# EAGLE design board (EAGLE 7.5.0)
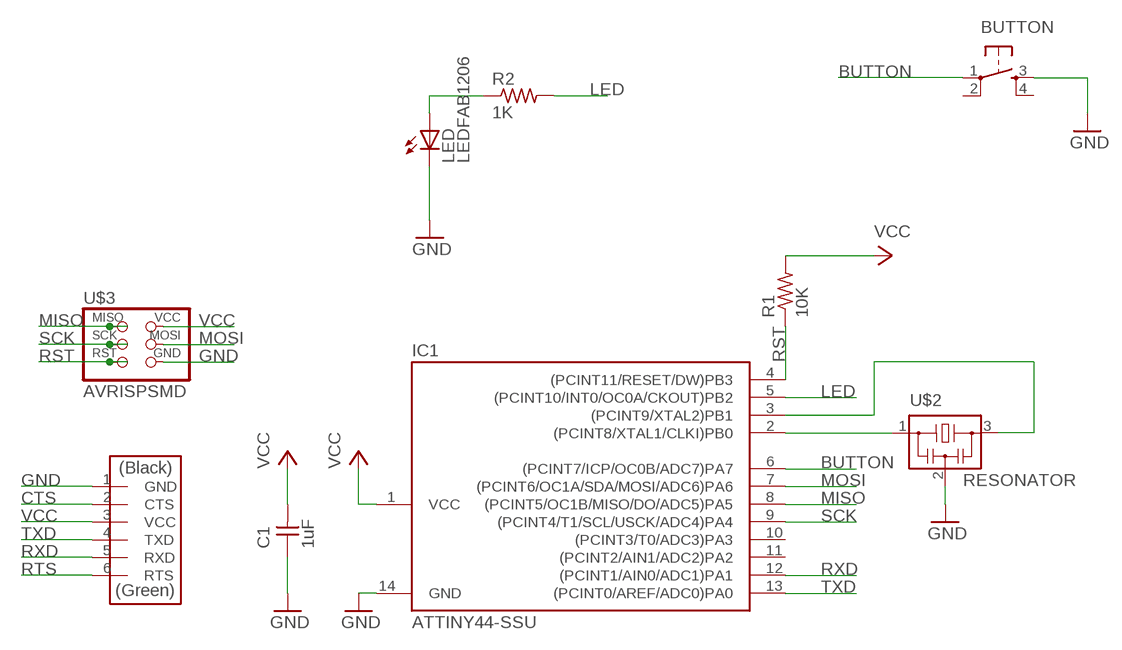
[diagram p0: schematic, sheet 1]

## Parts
BUTTON  6MM_SWITCH6MM_SWITCH  [6MM_SWITCH]
C1  1uF  CAP-UNPOLARIZED  [C1206]
IC1  ATTINY44-SSU  [SOIC14]
LED  LEDFAB1206  [LED1206FAB]
R1  10K  RES-US1206FAB  [R1206FAB]
R2  1K  RES-US1206FAB  [R1206FAB]
U$2  RESONATOR  [EFOBM]
U$3  AVRISPSMD  [2X03SMD]
U$4  FTDI-SMD-HEADER  [1X06SMD]

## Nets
BUTTON: BUTTON.1(P) IC1.6((PCINT7/ICP/OC0B/ADC7)PA7)
CTS: U$4.2(CTS)
GND: BUTTON.3(S) C1.1 IC1.14(GND) LED.2(C) U$2.2 U$3.6(GND) U$4.1(GND)
LED: IC1.5((PCINT10/INT0/OC0A/CKOUT)PB2) R2.2
MISO: IC1.8((PCINT5/OC1B/MISO/DO/ADC5)PA5) U$3.1(MISO)
MOSI: IC1.7((PCINT6/OC1A/SDA/MOSI/ADC6)PA6) U$3.4(MOSI)
N$1: IC1.3((PCINT9/XTAL2)PB1) U$2.3
N$2: IC1.2((PCINT8/XTAL1/CLKI)PB0) U$2.1
N$3: LED.1(A) R2.1
RST: IC1.4((PCINT11/RESET/DW)PB3) R1.1 U$3.5(RST)
RTS: U$4.6(RTS)
RXD: IC1.12((PCINT1/AIN0/ADC1)PA1) U$4.5(RXD)
SCK: IC1.9((PCINT4/T1/SCL/USCK/ADC4)PA4) U$3.3(SCK)
TXD: IC1.13((PCINT0/AREF/ADC0)PA0) U$4.4(TXD)
VCC: C1.2 IC1.1(VCC) R1.2 U$3.2(VCC) U$4.3(VCC)
Unconnected: BUTTON.2(P1) BUTTON.4(S1) IC1.10((PCINT3/T0/ADC3)PA3) IC1.11((PCINT2/AIN1/ADC2)PA2)

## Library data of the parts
BUTTON = fab:6MM_SWITCH: OMRON SWITCH
C1 = fab:CAP-UNPOLARIZED
IC1 = fab:ATTINY44
LED = fab:LED: LED
R1 R2 = fab:RES-US: Resistor (US Symbol)
U$2 = fab:RESONATOR
U$3 = fab:AVRISP
U$4 = fab:FTDI-SMD-HEADER

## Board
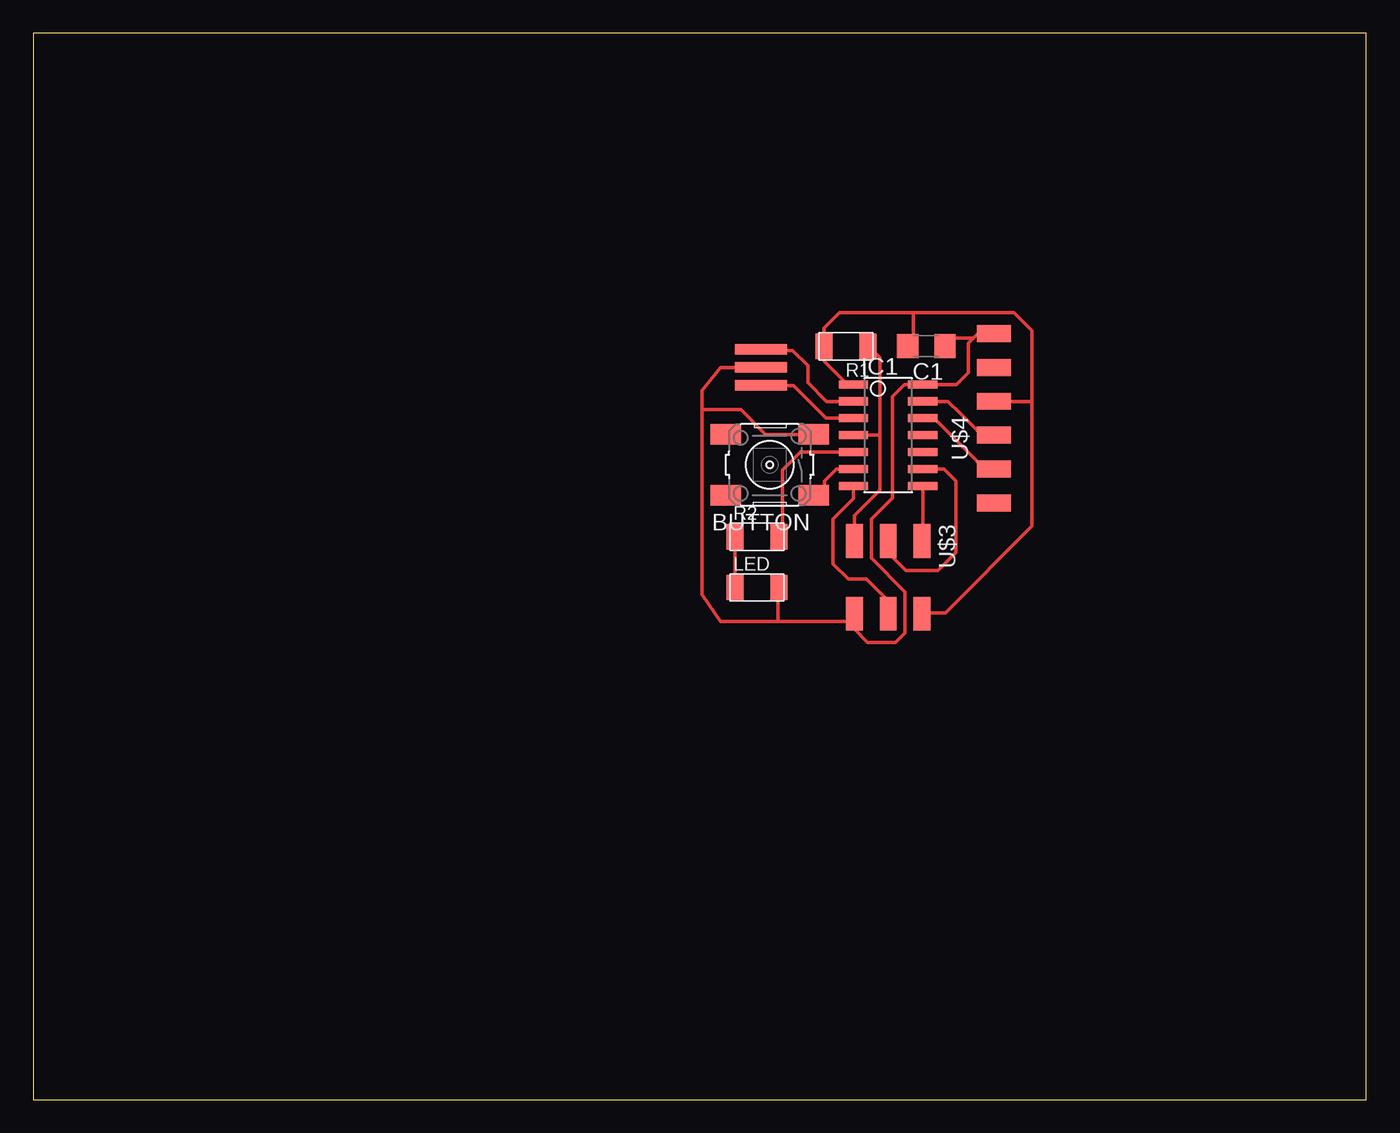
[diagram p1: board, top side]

Size 100 x 80 mm. Coordinates in mm from the lower left corner, seen from the top.
Outline: 0,0 100,0 100,80 0,80 0,0
Copper layers (1*16): Top 0.035mm / dielectric 1.5mm / Bottom 0.035mm
Design rules "default": minimum track width 10mil, minimum drill 24mil, track to track 8mil, track to pad 8mil, pad to pad 8mil, via to via 8mil, smd to smd 8mil, copper to edge 40mil, drill to drill 8mil, minimum pad ring 10mil, minimum via ring 8mil, stop-mask expansion 4mil, vias tented up to drill 0mil, thermal gap 10mil

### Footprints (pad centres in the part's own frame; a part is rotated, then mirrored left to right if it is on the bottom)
6MM_SWITCH = smd 2.286 x 1.524: 1 -3.302,2.286; 2 3.302,2.286; 3 -3.302,-2.286; 4 3.302,-2.286
C1206 = smd 1.6 x 1.8: 1 -1.4,0; 2 1.4,0
SOIC14 = smd 0.61 x 2.21: 1 -3.81,-2.603; 2 -2.54,-2.603; 3 -1.27,-2.603; 4 0,-2.603; 5 1.27,-2.603; 6 2.54,-2.603; 7 3.81,-2.603; 8 3.81,2.603; 9 2.54,2.603; 10 1.27,2.603; 11 0,2.603; 12 -1.27,2.603; 13 -2.54,2.603; 14 -3.81,2.603
LED1206FAB = smd 1.27 x 1.905: 1 -1.651,0; 2 1.651,0
R1206FAB = smd 1.27 x 1.905: 1 -1.651,0; 2 1.651,0
EFOBM = smd 0.8 x 3.9: 1 -1.35,0; 2 0,0; 3 1.35,0
2X03SMD = smd 2.54 x 1.27: 1 -2.54,2.54; 2 2.92,2.54; 3 -2.54,0; 4 2.92,0; 5 -2.54,-2.54; 6 2.92,-2.54
1X06SMD = smd 2.54 x 1.27: 1 0,6.35; 2 0,3.81; 3 0,1.27; 4 0,-1.27; 5 0,-3.81; 6 0,-6.35

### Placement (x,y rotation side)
BUTTON  55.24,47.62 180 top
C1  66.99,56.52 180 top
IC1  64.14,49.85 270 top
LED  54.29,38.42 0 top
R1  60.96,56.52 180 top
R2  54.29,42.23 0 top
U$2  54.61,54.93 270 top
U$3  64.14,39.37 270 top
U$4  72.07,51.12 0 top

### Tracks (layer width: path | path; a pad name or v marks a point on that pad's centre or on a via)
BUTTON
  Top 0.254: BUTTON.1 59.37,45.34 59.37,46.41 60.27,47.31 IC1.6
GND
  Top 0.254: U$2.2 51.56,54.93 50.16,53.21 50.16,51.75 | 50.16,51.75 50.16,37.89 51.54,35.88 55.88,35.88 | 55.88,35.88 61.59,35.88 U$3.6 61.59,35.29 62.6,34.29 64.69,34.29 65.41,35 65.41,38.1 62.87,40.64 62.87,43.55 64.45,45.14 64.45,52.76 65.35,53.66 IC1.14 69.27,53.66 70.17,54.56 70.17,56.76 70.52,57.11 | LED.2 55.88,38.42 55.88,35.88 | BUTTON.3 54.93,49.91 53.09,51.75 50.16,51.75 | U$4.1 70.88,57.47 70.52,57.11 | C1.1 68.26,56.52 68.26,57.15 70.52,57.15 70.52,57.11
LED
  Top 0.254: R2.2 56.2,42.23 56.2,47.23 57.55,48.58 IC1.5
MISO
  Top 0.254: U$3.1 66.74,41.91 IC1.8
MOSI
  Top 0.254: U$3.4 64.14,37.43 62.52,39.05 61.15,39.05 60.01,40.2 60.01,43.56 61.53,45.09 IC1.7
N$1
  Top 0.254: U$2.3 57.02,53.58 57.47,53.13 59.48,51.12 IC1.3
N$2
  Top 0.254: IC1.2 59.52,52.39 58.1,53.81 58.1,55.05 56.96,56.2 54.61,56.2 U$2.1
N$3
  Top 0.254: R2.1 LED.1
RST
  Top 0.254: 61.91,41.91 U$3.5 61.59,43.81 63.5,45.72 63.5,49.85 | 61.28,49.85 IC1.4 63.5,49.85 | R1.1 63.5,55.69 63.5,49.85
RXD
  Top 0.254: U$4.5 71.39,47.31 68.58,50.11 67.58,51.12 IC1.12
SCK
  Top 0.254: IC1.9 68.32,47.31 69.22,46.41 69.22,41.03 67.87,39.69 65.46,39.69 64.45,40.69 64.45,41.59 64.14,41.59 U$3.3
TXD
  Top 0.254: U$4.4 71.17,49.85 69.53,51.49 68.63,52.39 IC1.13
VCC
  Top 0.254: 66.04,59.05 60.49,59.05 59.31,57.87 R1.2 59.37,56.52 59.37,55.37 61.08,53.66 IC1.1 | 66.04,59.05 73.58,59.05 74.93,57.71 74.93,52.39 | U$4.3 74.93,52.39 | 74.93,52.39 74.93,43.03 68.42,36.51 66.67,36.51 U$3.2 | C1.2 66.04,56.52 66.04,59.05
